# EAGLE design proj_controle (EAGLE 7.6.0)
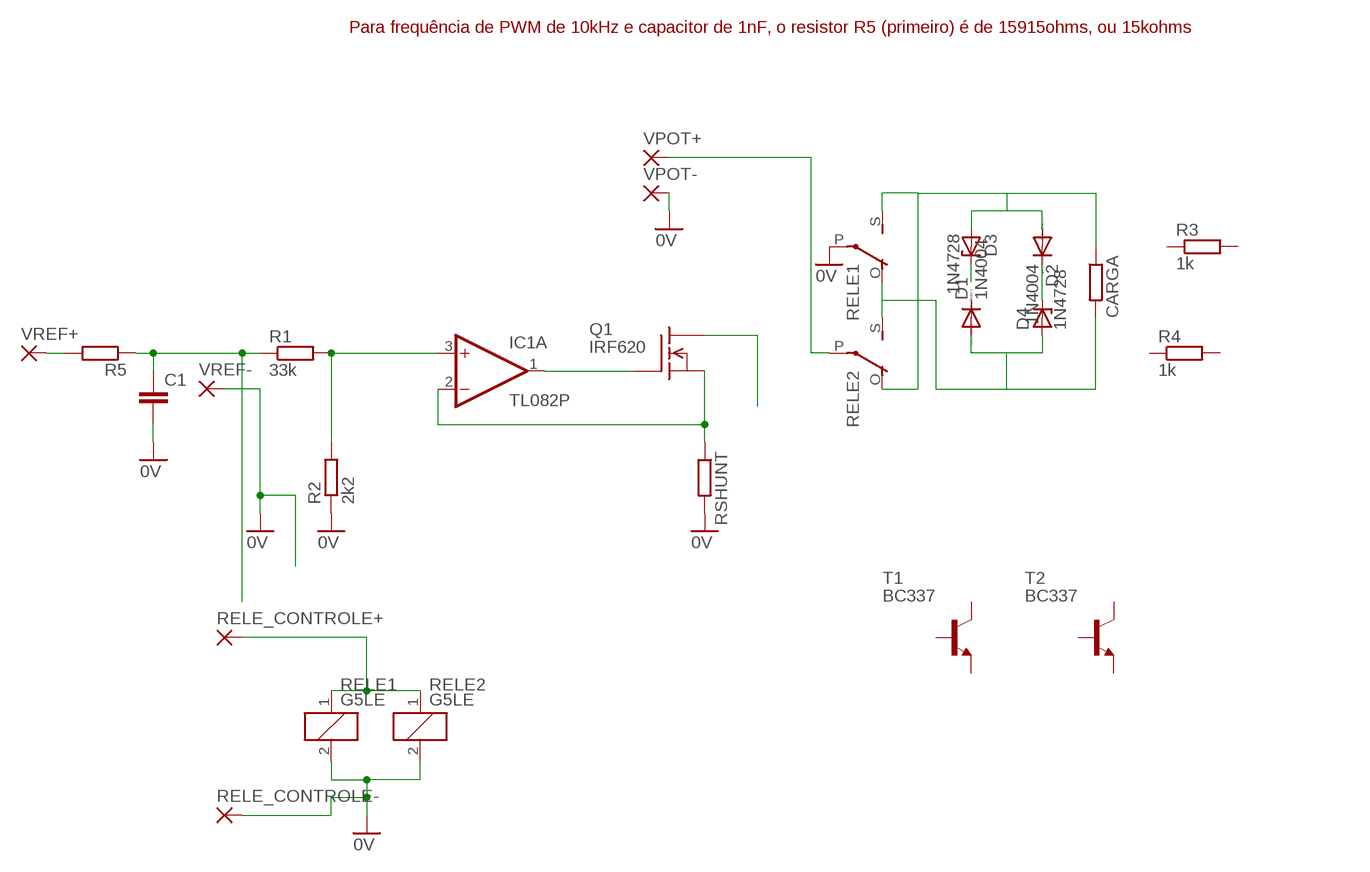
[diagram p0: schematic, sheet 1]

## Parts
C1  C-EU050-025X075  [C050-025X075]
CARGA  R-EU_0207/10  [0207/10]
D1  1N4004  [DO41-10]
D2  1N4004  [DO41-10]
D3  1N4728  [DO41Z10]
D4  1N4728  [DO41Z10]
IC1  TL082P  [DIL08]
Q1  IRF620  [TO220]
R1  33k  R-EU_0207/10  [0207/10]
R2  2k2  R-EU_0207/10  [0207/10]
R3  1k  R-EU_0207/10  [0207/10]
R4  1k  R-EU_0207/10  [0207/10]
R5  R-EU_0207/10  [0207/10]
RELE1  G5LE  [G5LE]
RELE2  G5LE  [G5LE]
RELE_CONTROLE+  3,17/1,1  [3,17/1,1]
RELE_CONTROLE-  3,17/1,1  [3,17/1,1]
RSHUNT  R-EU_0617/22  [0617/22]
T1  BC337  [TO92]
T2  BC337  [TO92]
VPOT+  3,17/1,1  [3,17/1,1]
VPOT-  3,17/1,1  [3,17/1,1]
VREF+  3,17/1,1  [3,17/1,1]
VREF-  3,17/1,1  [3,17/1,1]

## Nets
0V: C1.2 R2.1 RELE1.2 RELE1.P(2:P) RELE2.2 RELE_CONTROLE-.1(P) RSHUNT.2 VPOT-.1(P) VREF-.1(P)
N$1: D3.C
N$2: IC1.3(A:+IN) R1.2 R2.2
N$3: IC1.1(A:OUT) Q1.1(G)
N$4: IC1.2(A:-IN) Q1.3(S) RSHUNT.1
N$5: C1.1 R1.1 R5.1
N$6: R5.2 VREF+.1(P)
N$7: D2.C D4.C
N$8: Q1.2(D)
N$9: CARGA.2 D1.A D4.A RELE1.O(2:O) RELE2.S(2:S)
N$10: RELE2.P(2:P) VPOT+.1(P)
N$11: CARGA.1 D2.A D3.A RELE1.S(2:S) RELE2.O(2:O)
N$15: RELE1.1 RELE2.1 RELE_CONTROLE+.1(P)
Unconnected: D1.C IC1.5(B:+IN) IC1.6(B:-IN) IC1.7(B:OUT) R3.1 R3.2 R4.1 R4.2 T1.1(E) T1.2(B) T1.3(C) T2.1(E) T2.2(B) T2.3(C)

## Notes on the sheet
- Para frequência de PWM de 10kHz e capacitor de 1nF, o resistor R5 (primeiro) é de 15915ohms, ou 15kohms

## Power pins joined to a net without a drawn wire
V+: IC1.8(P:V+)
V-: IC1.4(P:V-)

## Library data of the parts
C1 = rcl:C-EU: CAPACITOR, European symbol
CARGA R1-R5 = rcl:R-EU_: RESISTOR, European symbol
D1 D2 = diode:1N4004: DIODE
D3 D4 = diode:1N4728: Z DIODE
IC1 = linear:TL082: OP AMP Data sheet; DATA_SHEET: <a href="http://www.ti.com/lit/ds/symlink/tl084a.pdf"> Data sheet </a>
Q1 = transistor-fet:IRF620: N-Channel Enhancement MOSFET (HEXFET); 200V; 5,2A; 0,8Ohm
RELE1 RELE2 = relay:G5LE: RELAY 1 x switch, 10 A/120 V AC, 8 A/30 V DC, Omron; OC_FARNELL: unknown; OC_NEWARK: unknown
RELE_CONTROLE+ RELE_CONTROLE- VPOT+ VPOT- VREF+ VREF- = wirepad:3,17/1,1: THROUGH-HOLE PAD
RSHUNT = resistor:R-EU_: RESISTOR, European symbol
T1 T2 = transistor:BC337: NPN TRANSISTOR

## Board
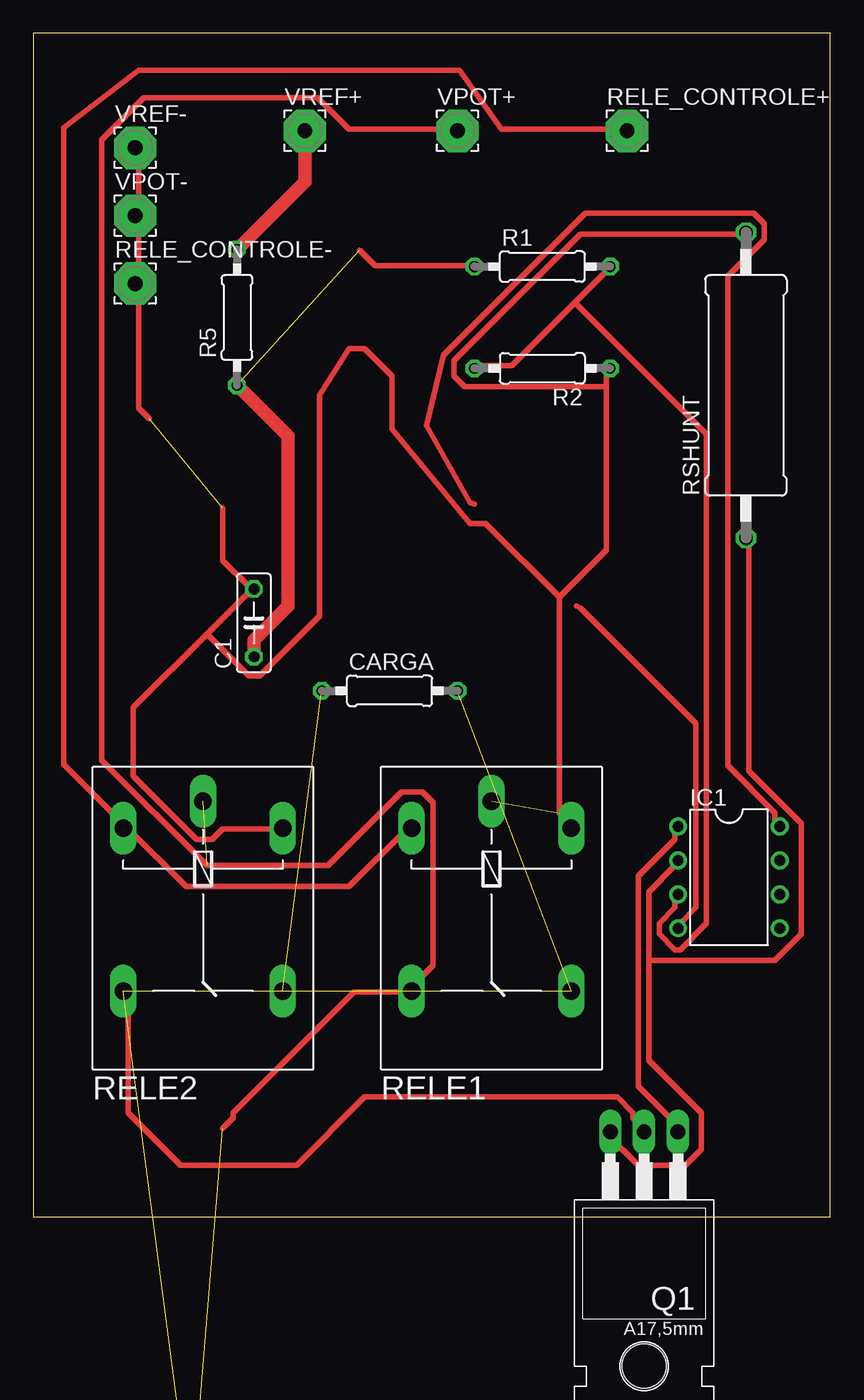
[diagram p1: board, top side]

Size 59.67 x 88.57 mm. Coordinates in mm from the lower left corner, seen from the top.
Outline: 0,0 59.67,0 59.67,88.57 0,88.57 0,0
Copper layers (1*16): Top 0.035mm / dielectric 1.5mm / Bottom 0.035mm
Design rules "default *": minimum track width 16mil, minimum drill 24mil, track to track 15mil, track to pad 15mil, pad to pad 15mil, via to via 15mil, smd to smd 8mil, copper to edge 40mil, drill to drill 8mil, minimum pad ring 10mil, minimum via ring 8mil, stop-mask expansion 4mil, vias tented up to drill 0mil, thermal gap 10mil

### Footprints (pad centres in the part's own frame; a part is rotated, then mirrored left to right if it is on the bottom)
C050-025X075 = drill 0.813 octagon: 1 -2.54,0; 2 2.54,0
0207/10 = drill 0.813 octagon: 1 -5.08,0; 2 5.08,0
DO41-10 = drill 1.118: A 5.08,0; C -5.08,0
DO41Z10 = drill 1.118: A 5.08,0; C -5.08,0
DIL08 = drill 0.813 pad 1.27: 1 -3.81,-3.81; 2 -1.27,-3.81; 3 1.27,-3.81; 4 3.81,-3.81; 5 3.81,3.81; 6 1.27,3.81; 7 -1.27,3.81; 8 -3.81,3.81
TO220 = drill 1.118 long: 1 -2.54,-6.35; 2 0,-6.35; 3 2.54,-6.35 | hole 3.302: 0,11.176
G5LE = drill 1.321 long: 1 -7.493,-5.969; 2 -7.493,5.969; O 4.699,5.969; P -9.525,0; S 4.699,-5.969
3,17/1,1 = drill 1.118 pad 3.175 octagon: 1 0,0
0617/22 = drill 1.016 octagon: 1 -11.43,0; 2 11.43,0
TO92 = drill 0.813 octagon: 1 1.27,0; 2 0,1.905; 3 -1.27,0

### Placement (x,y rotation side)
C1  16.51,44.45 90 top
CARGA  26.67,39.37 0 top
D1  not placed on the board
D2  not placed on the board
D3  not placed on the board
D4  not placed on the board
IC1  52.07,25.4 270 top
Q1  45.72,0 180 top
R1  38.1,71.12 0 top
R2  38.1,63.5 180 top
R3  not placed on the board
R4  not placed on the board
R5  15.24,67.31 90 top
RELE1  34.29,21.59 270 top
RELE2  12.7,21.59 270 top
RELE_CONTROLE+  44.45,81.28 0 top
RELE_CONTROLE-  7.62,69.85 0 top
RSHUNT  53.34,62.23 90 top
T1  not placed on the board
T2  not placed on the board
VPOT+  31.75,81.28 0 top
VPOT-  7.62,74.93 0 top
VREF+  20.32,81.28 0 top
VREF-  7.62,80.01 0 top

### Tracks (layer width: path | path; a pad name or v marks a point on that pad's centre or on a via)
0V  (2 unrouted)
  Top 0.406: 42.91,62.12 42.91,49.91 39.37,46.37 | 42.91,62.12 42.91,63.3 R2.1 | 39.37,46.37 39.37,30.23 40.16,29.44 RELE1.2 | 42.91,62.12 32.28,62.12 31.5,62.9 31.5,64.08 40.95,73.53 53.15,73.53 RSHUNT.2 | VREF-.1 7.87,79.83 7.87,75.11 VPOT-.1 7.87,74.71 7.87,69.99 RELE_CONTROLE-.1 7.87,69.6 7.87,60.54 8.66,59.75 | 14.17,53.06 14.17,49.12 16.14,47.15 C1.2 16.14,46.76 12.99,43.61 | 12.99,43.61 7.48,38.1 7.48,32.98 12.21,28.26 13.39,28.26 14.17,29.05 18.5,29.05 RELE2.2 | 39.37,46.37 33.86,51.88 32.68,51.88 26.86,58.97 26.86,62.9 24.8,64.96 23.62,64.96 21.44,61.51 21.44,44.97 16.93,40.46 16.14,40.46 12.99,43.61
N$2
  Top 0.406: 40.55,68.42 42.91,70.78 R1.2 | 40.55,68.42 35.83,63.69 33.07,63.69 R2.2 | 40.55,68.42 50.39,58.57 50.39,21.96 48.42,19.99 48.03,19.99 46.85,21.17 46.85,21.96 48.03,23.14 48.03,23.93 IC1.3
N$3
  Top 0.406: IC1.1 48.03,29.05 48.03,28.26 45.28,25.5 45.28,9.75 48.42,6.6 Q1.1
N$4
  Top 0.406: 46.06,19.2 46.06,11.72 50,7.79 50,5.03 48.82,3.85 45.28,3.85 42.91,6.21 Q1.3 | 46.06,19.2 46.06,24.32 48.03,26.29 IC1.2 | 46.06,19.2 55.51,19.2 57.48,21.17 57.48,29.44 53.54,33.38 53.54,50.7 RSHUNT.1
N$5  (1 unrouted)
  Top 0.406: 24.41,72.35 25.59,71.17 32.68,71.17 R1.1
  Top 1.016: C1.1 16.51,43.18 19.05,45.72 19.05,58.42 R5.1
N$6
  Top 1.016: VREF+.1 20.32,77.47 R5.2
N$7  (1 unrouted)
N$8
  Top 0.406: 7.09,16.84 7.09,7.79 11.02,3.85 19.68,3.85 24.8,8.97 43.7,8.97 44.88,7.79 44.88,7.39 45.67,6.6 Q1.2
N$9  (4 unrouted)
N$10  (1 unrouted)
  Top 0.406: 28.35,17.23 29.92,18.81 29.92,31.01 29.13,31.8 27.56,31.8 22.05,26.29 12.99,26.29 5.12,34.16 5.12,80.62 8.27,83.77 21.26,83.77 23.62,81.41 31.5,81.41 VPOT+.1
N$11  (4 unrouted)
  Top 0.406: 14.17,6.6 14.96,7.39 14.96,7.79 24.02,16.84 27.95,16.84 RELE1.S
N$15
  Top 0.406: RELE1.1 27.95,29.05 23.62,24.71 11.42,24.71 7.09,29.05 RELE2.1 6.69,29.44 2.27,33.86 2.27,81.5 7.87,85.83 31.89,85.83 35.04,81.41 44.09,81.41 RELE_CONTROLE+.1
V+
  Top 0.406: IC1.8 55.51,29.44 55.51,30.23 51.97,33.77 51.97,70.38 54.72,73.14 54.72,74.32 53.94,75.11 41.34,75.11 30.71,64.48 29.44,59.23 32.68,53.45 33.02,53.34
V-
  Top 0.406: IC1.4 48.42,21.96 49.61,23.14 49.61,36.92 40.95,45.58 40.64,45.72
